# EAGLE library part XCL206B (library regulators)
Non-Isolated PoL Module DC DC Converter 1 Output 1.8V 600mA 2V - 6V Input
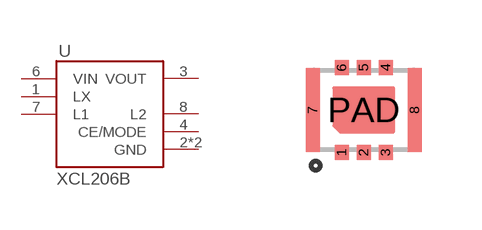
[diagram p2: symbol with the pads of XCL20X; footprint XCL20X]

Designator prefix U

## XCL206B" (DIGIKEY: 893-1406-2-ND; MPN: XCL206B183CR-G)  [XCL20X]
1  LX
2  GND
3  VOUT
4  CE/MODE
5  GND
6  VIN
7  L1
8  L2

## Footprint XCL20X (pad centres in mm)
smd 0.35 x 0.375: 1 -0.55,-1.062; 2 0,-1.062; 3 0.55,-1.062; 4 0.55,1.062; 5 0,1.062; 6 -0.55,1.062
smd 0.35 x 2.1: 7 -1.275,0; 8 1.275,0
smd 1.5 x 0.9: PAD 0,0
